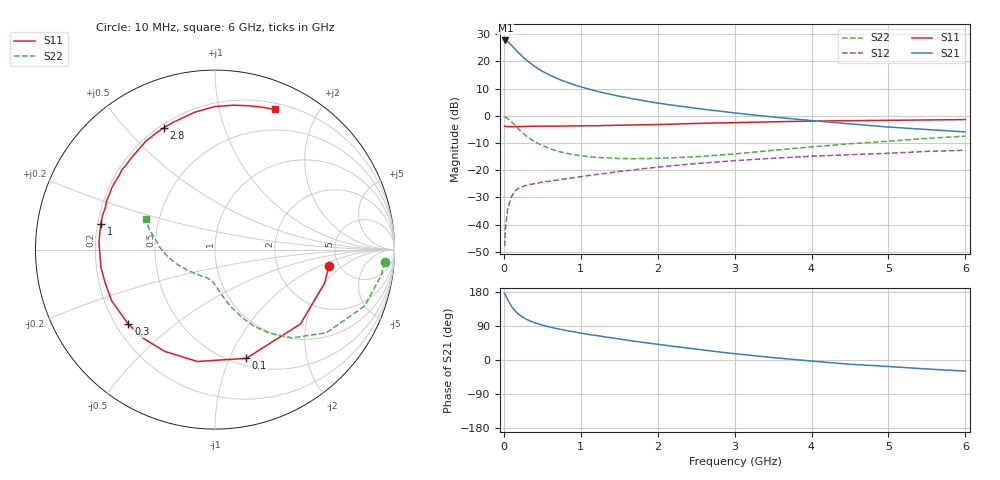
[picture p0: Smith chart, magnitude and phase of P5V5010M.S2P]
! SIEMENS Small Signal Semiconductors
! BFP183
! Si NPN RF Bipolar Junction Transistor in SOT143
! VCE = 0.5 V  IC = 10 mA
! Common Emitter S-Parameters:  March  1996
# GHz  S  MA  R  50
!  f  S11  S21  S12  S22
! GHz  MAG  ANG  MAG  ANG  MAG  ANG  MAG  ANG
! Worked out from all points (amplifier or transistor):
!   36 points, 10 MHz to 6 GHz, reference 50 ohm
!   highest |S21| = 27.7 dB at 20 MHz (marker M1)
!   |S21| within 3 dB of that: start of sweep to 141 MHz
!   unconditionally stable (mu >= 1): 828.7 MHz to end of sweep
!   at 250 MHz: K = 0.39, MSG = 23.8 dB, |S12| = -26.0 dB
!   at 1.4 GHz: K = 1.26, MAG = 11.3 dB, |S12| = -20.9 dB
!   at 6 GHz: K = 1.18, MAG = 0.8 dB, |S12| = -12.7 dB
!   S11 on the Smith chart (normalised r, x): 10 MHz: 4.14, -1.30; 100 MHz: 0.57, -1.15; 300 MHz: 0.25, -0.35; 1 GHz: 0.21, +0.11; 2.8 GHz: 0.22, +0.64; 6 GHz: 0.26, +1.49
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0.01  0.6414 -8.3  24.16 175.9  0.004 85.5  0.9475 -4.2
0.02  0.6383 -17.3  24.2 171.7  0.0085 81.0  0.9385 -8.5
0.05  0.6312 -41.1  22.99 158.9  0.0191 73.7  0.8924 -20.5
0.1  0.6305 -74.0  19.73 141.9  0.0329 57.5  0.7745 -36.8
0.15  0.6311 -99.0  16.61 128.8  0.0419 48.3  0.6524 -48.9
0.2  0.6326 -116.4  14.01 119.5  0.0471 42.5  0.5536 -57.1
0.25  0.6356 -129.2  11.91 112.3  0.0501 38.9  0.4774 -63.1
0.3  0.637 -139.2  10.34 106.8  0.0531 36.5  0.4157 -67.6
0.4  0.6428 -153.7  8.065 98.2  0.0565 34.2  0.3331 -74.2
0.5  0.6395 -163.6  6.555 92.1  0.0601 33.2  0.2834 -78.6
0.6  0.6434 -171.5  5.569 86.7  0.0628 33.8  0.2486 -82.2
0.7  0.6415 -177.6  4.769 82.3  0.0657 34.1  0.223 -85.3
0.8  0.6473 176.9  4.219 78.2  0.0689 34.8  0.2058 -88.0
1  0.6514 167.4  3.399 71.1  0.0758 35.9  0.1843 -92.7
1.1  0.6549 163.2  3.103 67.6  0.0795 36.5  0.1774 -95.2
1.5  0.6701 149.3  2.284 55.3  0.0943 37.5  0.1635 -104.8
2.2  0.6999 128.1  1.557 36.1  0.121 35.3  0.1688 -124.5
2.8  0.7365 112.7  1.218 21.1  0.1421 31.2  0.1898 -141.3
3.5  0.7737 98.4  0.948 6.3  0.1653 25.9  0.2314 -160.3
4.5  0.8111 82.6  0.708 -11.2  0.1922 17.5  0.3056 178.1
5.5  0.8357 71.7  0.558 -23.7  0.2208 10.1  0.3833 163.0
6  0.8501 66.7  0.504 -29.4  0.2318 5.6  0.4216 156.3
